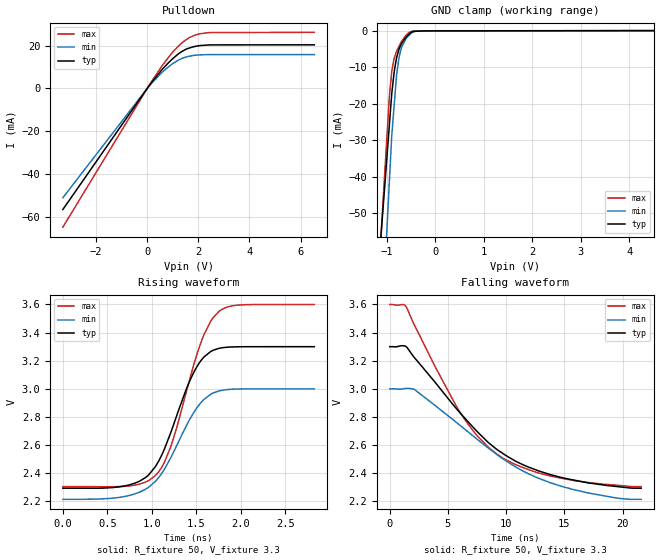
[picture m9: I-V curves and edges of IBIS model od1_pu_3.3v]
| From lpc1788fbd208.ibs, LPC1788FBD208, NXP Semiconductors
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[Model]   od1_pu_3.3v
Model_type I/O_open_drain
Vinl=8.000E-01
Vinh=2.000E+00
Vref=3.300E+00
Rref=2.000E+03
Cref=0.000E+00
Vmeas=1.650E+00
C_comp   1.240E-12   1.180E-12   1.300E-12
[Voltage Range]   3.300E+00   3.000E+00   3.600E+00
[POWER Clamp Reference]   3.300E+00   3.000E+00   3.600E+00
[GND Clamp Reference]   0.000E+00   0.000E+00   0.000E+00
[Pullup Reference]   3.300E+00   3.000E+00   3.600E+00
[Pulldown Reference]   0.000E+00   0.000E+00   0.000E+00
[Temperature Range]   25   85   -40
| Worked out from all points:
|   slope of the pulldown table from 0 to 0.495 V, typ, clamps not added: 65.7 ohm
|   GND clamp passes 1 mA (typ) near -0.54 V on its own axis
|   rising waveform, R_fixture 50, V_fixture 3.3: 20-80 % time 373ps typ, 403ps min, 362ps max; typ from 2.29 V to 3.3 V
|   falling waveform, R_fixture 50, V_fixture 3.3: 20-80 % time 7.24ns typ, 8.09ns min, 5.99ns max; typ from 3.3 V to 2.29 V
[GND Clamp]
-3.3V     -438.5mA   -646.2mA   -539.2mA
-950mV    -26.12mA   -41.76mA   -18.22mA
-900mV    -17.35mA   -28.9mA    -11.22mA
-850mV    -11.36mA   -20.52mA   -7.6mA
-800mV    -7.442mA   -12.15mA   -5.625mA
-750mV    -5.079mA   -7.409mA   -4.294mA
-700mV    -3.596mA   -4.64mA    -2.964mA
-600mV    -1.693mA   -2.032mA   -1.181mA
-500mV    -488.5uA   -682uA     -233.7uA
-400mV    -173.2uA   -129.9uA   -101.2uA
-200mV    -62.56uA   -47.1uA    -77.07uA
6.6V      35.04uA    32.39uA    35.06uA
[Pulldown]
-3.3V     -56.5mA    -51.02mA   -64.74mA
133mV     2.157mA    1.865mA    2.546mA
552.2mV   8.383mA    7.138mA    10.03mA
791.7mV   11.49mA    9.679mA    13.86mA
1.011V    14.03mA    11.69mA    17.12mA
1.41V     17.6mA     14.25mA    21.79mA
1.65V     18.89mA    15.04mA    23.71mA
1.869V    19.61mA    15.52mA    24.88mA
2.389V    20.29mA    15.78mA    26.03mA
6.54V     20.37mA    15.82mA    26.19mA
[Rising Waveform]
R_fixture = 50
V_fixture = 3.3
V_fixture_min = 3
V_fixture_max = 3.6
0s        2.293V     2.214V     2.304V
725ps     2.314V     2.239V     2.308V
925ps     2.368V     2.285V     2.336V
1.041ns   2.448V     2.343V     2.384V
1.214ns   2.692V     2.512V     2.592V
1.487ns   3.136V     2.848V     3.206V
1.586ns   3.227V     2.925V     3.386V
1.76ns    3.289V     2.986V     3.553V
1.983ns   3.299V     2.999V     3.596V
2.825ns   3.3V       3V         3.6V
[Falling Waveform]
R_fixture = 50
V_fixture = 3.3
V_fixture_min = 3
V_fixture_max = 3.6
0s        3.3V       3V         3.6V
1.373ns   3.302V     3.003V     3.588V
2.147ns   3.219V     2.994V     3.449V
5.968ns   2.836V     2.745V     2.843V
7.541ns   2.694V     2.639V     2.663V
9.139ns   2.573V     2.536V     2.54V
11.5ns    2.458V     2.413V     2.438V
14.66ns   2.371V     2.309V     2.366V
19.05ns   2.309V     2.229V     2.317V
21.6ns    2.293V     2.214V     2.304V
[Ramp]
dV/dt_r   6.0392E-01/3.7240E-10   4.7144E-01/4.0290E-10   7.7735E-01/3.5950E-10
dV/dt_f   6.0392E-01/7.2206E-09   4.7144E-01/8.0847E-09   7.7735E-01/5.9653E-09
R_load = 50
